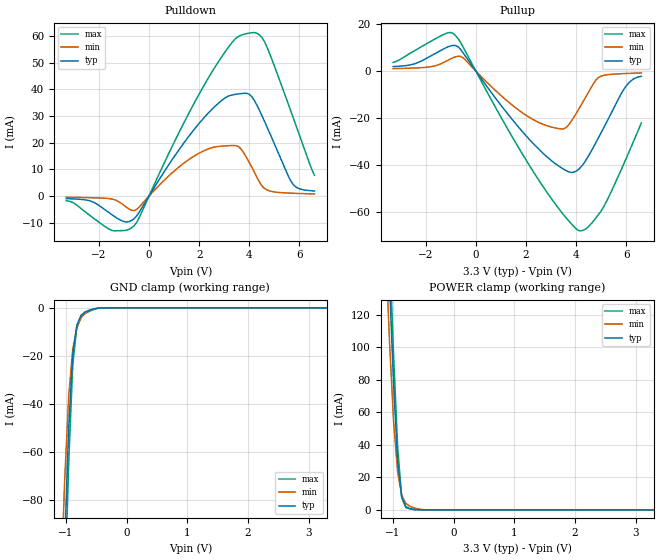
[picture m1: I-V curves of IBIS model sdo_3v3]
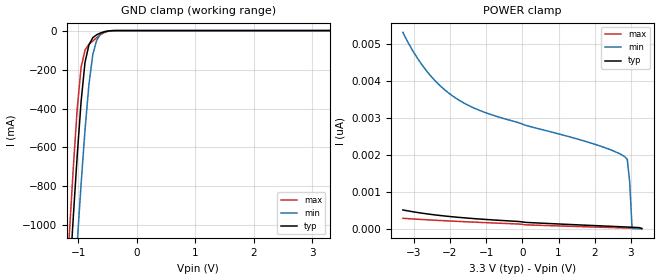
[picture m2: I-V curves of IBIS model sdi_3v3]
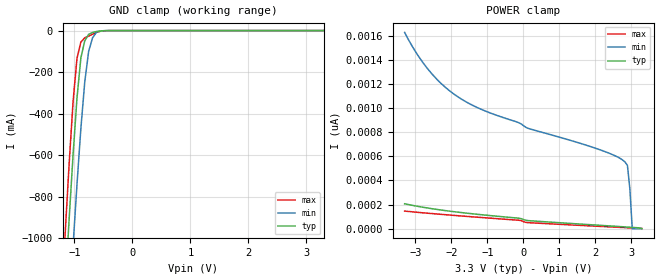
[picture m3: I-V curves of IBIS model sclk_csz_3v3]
| Texas Instruments Incorporated
| Marketing Part # : ADS112S14, ADS122S14
| Digital Voltage Range : 1.65V - 3.6V
| Package-type: QFN-RTE
| #pins/pkg drawing : QFN-16
[IBIS ver] 7.0
[File name]  ads112s14_ads122s14.ibs
[File Rev]  1.0
[Date]   05 27, 2026
[Source]
| Texas Instruments Incorporated.
| 12500 TI Blvd
| Dallas, TX -75243
[Notes] Revision History:
| Rev 1.0: 05/27/2026
| - Initial version of the model
| - Model generated from simulations in TISPICE/SPECTRE
| - C_comp although listed in numerical order of value are
|   obtained from varying PVT conditions. For PVT conditions for
|   each specific value refer the buffer description under
|   respective [Model]. IBIS model user is responsible for using
|   appropriate C_comp to simulate for Signal Integrity.
| - Warnings regarding combined Non-monotonicity of various models have been
|   reviewed and considered minor and can be ignored.
| - Model names with a trailing _1v8 contain the model for 1.8V operation.
| - Model names with a trailing _3v3 contain the model for 3.3V operation.
[Disclaimer]
| This model is designed as an aid for customers of Texas Instruments.
| TI and its licensors and suppliers make no warranties, either expressed
| or implied, with respect to this model, including the warranties of
| merchantability or fitness for a particular purpose. The model is
| provided solely on an "as is" basis. The entire risk as to its quality
| and performance is with the customer.
| This model is subject to change without notice. Texas Instruments
| Incorporated is not responsible for updating this model.
[Copyright]
(C) Copyright 2026 Texas Instruments Incorporated. All rights reserved.
| Component1 ADS1x2S14RTE
[Component] ADS1x2S14RTE
[Manufacturer] Texas Instruments Incorporated
[Package] |16 WQFN - RUK package
| variable   typ   min   max
R_pkg   50.000m   25.000m   100.000m
L_pkg   0.500nH   0.250nH   1.000nH
C_pkg   0.100pF   50.000fF   0.200pF
| pin number (pin name) mapping to model name
[Pin] signal_name   model_name   R_pin   L_pin   C_pin
1   AIN0   NC   NA   NA   NA
2   AIN1   NC   NA   NA   NA
3   AIN2   NC   NA   NA   NA
4   AIN3   NC   NA   NA   NA
5   AIN4   NC   NA   NA   NA
6   AIN5   NC   NA   NA   NA
7   AIN6   NC   NA   NA   NA
8   AIN7   NC   NA   NA   NA
9   CSn   input_sclk_csz NA   NA   NA
10   SDI   input_sdi   NA   NA   NA
11   SDO/DRDYn   output_sdo   NA   NA   NA
12   SCLK   input_sclk_csz NA   NA   NA
13   IOVDD   NC   NA   NA   NA
14   GND   NC   NA   NA   NA
15   AVDD   NC   NA   NA   NA
16   REFOUT   NC   NA   NA   NA
|***** end of component 1 definition
|***** Model Selections ********
|***** Power supply options *********
[Model Selector] input_sclk_csz
sclk_csz_1v8 input buffer at 1.8V operation.
sclk_csz_3v3 input buffer at 3.3V operation.
[Model Selector] input_sdi
sdi_1v8 input buffer at 1.8V operation.
sdi_3v3 input buffer at 3.3V operation.
[Model Selector] output_sdo
sdo_1v8 input buffer at 1.8V operation.
sdo_3v3 input buffer at 3.3V operation.
| Models and submodels in the file (6): sdo_3v3 (3-state), sdi_3v3 (Input), sclk_csz_3v3 (Input), sdo_1v8 (3-state), sdi_1v8 (Input), sclk_csz_1v8 (Input)
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|   Model sdo_3v3
[Model] sdo_3v3
Model_type 3-state
Polarity   Non-Inverting
Enable   Active-High
C_comp   1.600pF   0.800pF   3.200pF
[Temperature Range]   27.000   0.125k   -40.000
[Voltage Range]   3.300V   3.000V   3.600V
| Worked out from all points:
|   slope of the pulldown table from 0 to 0.495 V, typ, clamps not added: 66 ohm
|   slope of the pullup table from 0 to 0.495 V, typ, clamps not added: 67.5 ohm
|   GND clamp passes 1 mA (typ) near -0.62 V on its own axis
|   POWER clamp passes 1 mA (typ) near -0.73 V on its own axis
[Pulldown]
|Voltage   I(typ)   I(min)   I(max)
-3.3V     -921.7uA   -405.8uA   -1.69mA
-2.3V     -1.923mA   -604.1uA   -7.632mA
-1.5V     -6.81mA    -1.065mA   -12.76mA
-1V       -9.527mA   -3.431mA   -12.89mA
-600mV    -8.463mA   -5.469mA   -11.14mA
1.2V      17.4mA     10.93mA    23.87mA
2.4V      31.45mA    17.8mA     44.75mA
3.5V      38.19mA    18.85mA    59.37mA
4.1V      37.26mA    10.84mA    61.19mA
4.6V      28.17mA    2.918mA    57.98mA
5.7V      5.006mA    1.102mA    30.73mA
6.6V      1.917mA    825.3uA    7.836mA
[Pullup]
|Voltage   I(typ)   I(min)   I(max)
-3.3V     1.909mA    1.026mA    3.635mA
-1.8V     6.393mA    1.838mA    12.59mA
-900mV    10.91mA    5.705mA    15.93mA
-500mV    7.619mA    5.565mA    10.05mA
1.3V      -18.57mA   -13.14mA   -25.15mA
2.6V      -34.1mA    -22.25mA   -47.75mA
3.5V      -41.66mA   -24.52mA   -61.02mA
4.1V      -41.71mA   -16.24mA   -67.72mA
4.4V      -37.65mA   -10.72mA   -66.87mA
4.9V      -28.11mA   -2.651mA   -60.78mA
5.9V      -7.768mA   -1.08mA    -39.4mA
6.6V      -2.218mA   -801.1uA   -22.03mA
[GND_clamp]
|Voltage   I(typ)   I(min)   I(max)
-3.3V     -2.59A     -2.502A    -2.652A
-1.089V   -157.6mA   -120.4mA   -186.1mA
-1.022V   -98.84mA   -72.04mA   -121.8mA
-955mV    -50.01mA   -36.72mA   -64.56mA
-888mV    -19.26mA   -17.14mA   -23.69mA
-821mV    -7.27mA    -8.43mA    -7.991mA
-754mV    -3.173mA   -4.286mA   -3.815mA
-687mV    -1.72mA    -2.263mA   -2.418mA
-553mV    -529.3uA   -525.6uA   -783uA
-352mV    -4.762uA   -9.213uA   -3.113uA
3.3V      0A         0A         0A
[POWER_clamp]
|Voltage   I(typ)   I(min)   I(max)
-3.3V     2.665A     2.603A     2.705A
-1.122V   207mA      164.3mA    233.9mA
-1.055V   139.2mA    103.8mA    162.8mA
-988mV    77.62mA    54.62mA    95.67mA
-921mV    30.68mA    23.29mA    38.7mA
-854mV    7.996mA    9.08mA     7.692mA
-787mV    2.006mA    4.011mA    1.422mA
-720mV    730.5uA    2.191mA    566uA
-653mV    272.9uA    1.229mA    196.5uA
-452mV    2.05uA     53.78uA    272.3nA
3.3V      0A         0A         0A
[Ramp]
| variable   typ   min   max
dV/dt_r   1.856/0.281n   1.649/0.463n   2.057/0.186n
dV/dt_f   1.859/0.287n   1.638/0.486n   2.061/0.190n
R_load = 1.000k
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|   Model sdi_3v3
[Model] sdi_3v3
Model_type Input
Polarity   Non-Inverting
Enable   Active-High
Vinl =  0.990V
Vinh =  2.310V
C_comp   4.000pF   2.000pF   8.000pF
[Model Spec]
Vinh   2.310V   2.100V   2.520V
Vinl   0.990V   0.900V   1.080V
[Temperature Range]   27.000   0.125k   -40.000
[Voltage Range]   3.300V   3.000V   3.600V
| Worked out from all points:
|   GND clamp passes 1 mA (typ) near -0.45 V on its own axis
[GND_clamp]
|Voltage   I(typ)   I(min)   I(max)
-3.3V     -8.723A    -8.387A    -9.129A
-1.156V   -1.293A    -1.738A    -1.045A
-1.089V   -960.1mA   -1.411A    -708.5mA
-1.022V   -644.8mA   -1.093A    -404.7mA
-955mV    -364.9mA   -789.3mA   -188.6mA
-888mV    -163.1mA   -511mA     -100.6mA
-821mV    -73.83mA   -277.9mA   -70.24mA
-754mV    -36.19mA   -121.9mA   -53.48mA
-687mV    -21.39mA   -49.48mA   -36.14mA
-620mV    -12.11mA   -16.45mA   -20.6mA
-419mV    -359.2uA   -386.2uA   -458.5uA
3.3V      0A         0A         0A
[POWER_clamp]
|Voltage   I(typ)   I(min)   I(max)
-3.3V     507.3pA    5.32nA     281.2pA
-2.931V   443.4pA    4.67nA     257.6pA
-2.529V   387pA      4.138nA    234.7pA
-2.127V   341.3pA    3.749nA    213.8pA
-1.658V   297.9pA    3.43nA     191.4pA
-854mV    239.4pA    3.089nA    156.3pA
1.96V     84.46pA    2.301nA    44.84pA
2.831V    46.86pA    1.948nA    19.41pA
2.898V    43.87pA    1.882nA    17.49pA
2.965V    40.84pA    1.266nA    15.58pA
3.032V    37.74pA    0A         13.67pA
3.3V      0A         0A         6.068pA
|   Model sclk_csz_3v3
[Model] sclk_csz_3v3
Model_type Input
Polarity   Non-Inverting
Enable   Active-High
Vinl =  0.990V
Vinh =  2.310V
C_comp   1.000pF   0.500pF   2.000pF
[Model Spec]
Vinh   2.310V   2.100V   2.520V
Vinl   0.990V   0.900V   1.080V
[Temperature Range]   27.000   0.125k   -40.000
[Voltage Range]   3.300V   3.000V   3.600V
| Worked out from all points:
|   GND clamp passes 1 mA (typ) near -0.51 V on its own axis
[GND_clamp]
|Voltage   I(typ)   I(min)   I(max)
-3.3V     -8.28A     -7.976A    -8.613A
-1.156V   -1.224A    -1.66A     -963mA
-1.089V   -901.1mA   -1.342A    -635.5mA
-1.022V   -595.6mA   -1.034A    -340.6mA
-955mV    -324.7mA   -739.9mA   -133.8mA
-888mV    -131.2mA   -471mA     -55.55mA
-821mV    -49.34mA   -247.1mA   -34.58mA
-754mV    -18.25mA   -99.81mA   -26.62mA
-687mV    -9.129mA   -35.22mA   -17.27mA
-620mV    -4.609mA   -8.672mA   -8.764mA
-553mV    -1.974mA   -1.956mA   -3.638mA
3.3V      0A         0A         0A
[POWER_clamp]
|Voltage   I(typ)   I(min)   I(max)
-3.3V     206.4pA    1.628nA    145.8pA
-2.931V   184.9pA    1.438nA    135.4pA
-2.529V   165.2pA    1.28nA     124.9pA
-2.127V   148.3pA    1.163nA    114.9pA
-1.658V   131.3pA    1.064nA    103.8pA
151mV     66.54pA    830.8pA    49.54pA
1.96V     31pA       672.2pA    21.53pA
2.764V    15.84pA    569.7pA    9.561pA
2.898V    13.25pA    524.8pA    7.587pA
2.965V    11.94pA    331.4pA    6.602pA
3.032V    10.6pA     0A         5.618pA
3.3V      0A         0A         1.691pA
